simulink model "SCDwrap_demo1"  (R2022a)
settings: configuration reference "configurationSettings" (kept in a data dictionary, not in this file)
undefined symbols (not defined in the file or in its folder): signal1, signal2, signal3, signal4, signal6, signal7

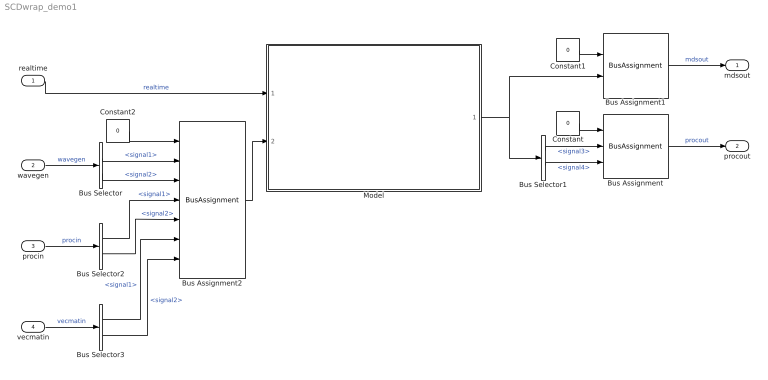
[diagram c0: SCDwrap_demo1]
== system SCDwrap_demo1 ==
  realtime : Inport  OutDataTypeStr=single
  wavegen : Inport  Port=2  OutDataTypeStr=Bus: WG0601bus
  procin : Inport  Port=3  OutDataTypeStr=Bus: procin
  vecmatin : Inport  Port=4  OutDataTypeStr=Bus: vecmatin
  Bus Assignment : BusAssignment  AssignedSignals=signal1,signal2
  Bus Assignment1 : BusAssignment  AssignedSignals=demo1
  Bus Assignment2 : BusAssignment  AssignedSignals=signal1,signal2,signal3,signal4,signal6,signal7
  Bus Selector : BusSelector  OutputSignals=signal1,signal2
  Bus Selector1 : BusSelector  OutputSignals=signal3,signal4
  Bus Selector2 : BusSelector  OutputSignals=proc02.signal1,proc02.signal2
  Bus Selector3 : BusSelector  OutputSignals=signal1,signal2
  Constant : Constant  Value=0  OutDataTypeStr=Bus: procout01
  Constant1 : Constant  Value=0  OutDataTypeStr=Bus: mdsout01
  Constant2 : Constant  Value=0  OutDataTypeStr=Bus: algo_demo1_inBus
  Model : ModelReference  ModelNameDialog=algo_demo1.slx  SimulationMode=Normal  ModelReferenceVersion=1.863  SimulationMode=Normal
  mdsout : Outport  OutDataTypeStr=Bus: mdsout01  VectorParamsAs1DForOutWhenUnconnected=off
  procout : Outport  Port=2  OutDataTypeStr=Bus: procout01  VectorParamsAs1DForOutWhenUnconnected=off
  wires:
  realtime/1 -> Model/1  "realtime"
  procin/1 -> Bus Selector2/1  "procin"
  wavegen/1 -> Bus Selector/1  "wavegen"
  Model/1 -> Bus Selector1/1, Bus Assignment1/2
  Bus Assignment/1 -> procout/1  "procout"
  Constant/1 -> Bus Assignment/1
  Constant1/1 -> Bus Assignment1/1
  Bus Assignment1/1 -> mdsout/1  "mdsout"
  Bus Selector/1 -> Bus Assignment2/2  "<signal1>"
  Constant2/1 -> Bus Assignment2/1
  Bus Assignment2/1 -> Model/2
  Bus Selector/2 -> Bus Assignment2/3  "<signal2>"
  Bus Selector2/1 -> Bus Assignment2/4  "<signal1>"
  Bus Selector2/2 -> Bus Assignment2/5  "<signal2>"
  Bus Selector1/1 -> Bus Assignment/2  "<signal3>"
  Bus Selector1/2 -> Bus Assignment/3  "<signal4>"
  vecmatin/1 -> Bus Selector3/1  "vecmatin"
  Bus Selector3/1 -> Bus Assignment2/6  "<signal1>"
  Bus Selector3/2 -> Bus Assignment2/7  "<signal2>"
